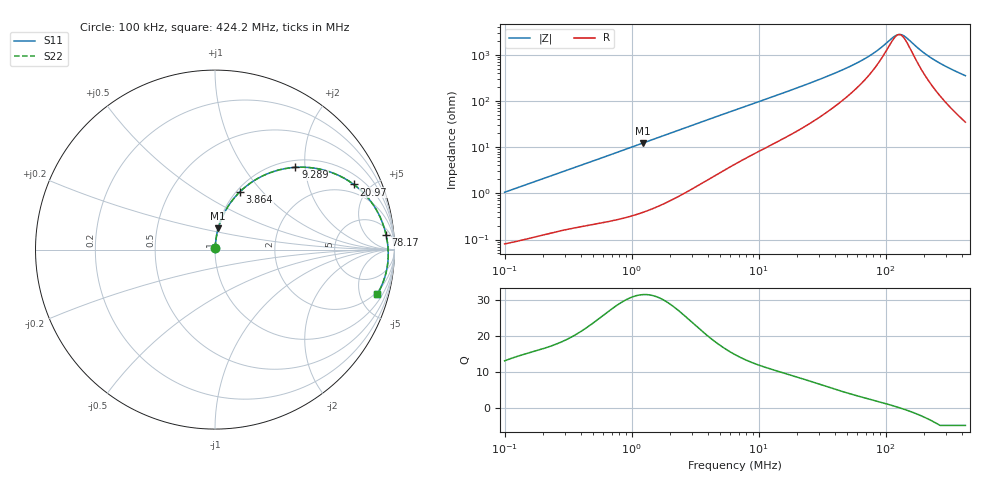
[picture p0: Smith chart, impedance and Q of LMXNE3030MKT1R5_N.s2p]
! LMXNE3030MKT1R5_N  S-PARAMETER MODEL  ( General Type )
! Model Generated by TAIYO YUDEN Corporation (https://www.yuden.co.jp/en/)
! Version 1.0
! TAIYO YUDEN Control No. 191023NI43SB-FBB
! Copyright(c) 2019 TAIYO YUDEN CO.,LTD. All Rights Reserved.
! Product Description (link to TY-COMPAS)
! https://ds.yuden.co.jp/TYCOMPAS/or/detail?pn=LMXNE3030MKT1R5NN&u=M
! Products Name : Inductors
! Characteristics :
!  Inductance : 1.5 uH , SRF(min) : 95 MHz , DC Resistance(max) : 0.066 Ohm
!  Rated Current : Saturation :1700 mA , Temp Rise : 1600 mA (40 degC)
!  Case Size : 3.0 x 3.0 / 0.118 x 0.118 [mm/inch] , Thickness : 1.2 / 0.047 [mm/inch]
!  (Conditions: Temperature = 25 degC , DC Bias Current/Voltage = 0A / 0V)
! External Node Assignments :
!  1  o---GGG---o  2
! GND o---------o GND
! Frequency Range : 0.1MHz  -  424.248007MHz  [ 402 STEP ]
# MHz S RI R 50
! Freq[MHz].  S11 Real  S11 Imag  S21 Real  S21 Imag  S12 Real  S12 Imag  S22 Real  S22 Imag
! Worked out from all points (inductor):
!   401 points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, 100 kHz to 424.2 MHz, reference 50 ohm
!   read as one part in series: L = 1.66 uH near 104.3 kHz
!   highest Q = 31.6 at 1.225 MHz (marker M1), where L = 1.59 uH
!   self-resonance near 127.2 MHz
!   S11 on the Smith chart (normalised r, x): 100 kHz: 1.00, +0.02; 3.864 MHz: 1.04, +0.76; 9.289 MHz: 1.14, +1.78; 20.97 MHz: 1.48, +3.96; 78.17 MHz: 10, +19; 424.2 MHz: 1.69, -6.98
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0.1  0.000914 0.0105  0.9991 -0.0105  0.9991 -0.0105  0.000914 0.0105
0.40516  0.00358 0.0408  0.9964 -0.0408  0.9964 -0.0408  0.00358 0.0408
1.225423  0.0184 0.1194  0.9816 -0.1194  0.9816 -0.1194  0.0184 0.1194
1.641544  0.0308 0.1574  0.9692 -0.1574  0.9692 -0.1574  0.0308 0.1574
2.598793  0.0703 0.2369  0.9297 -0.2369  0.9297 -0.2369  0.0703 0.2369
3.864414  0.1385 0.3218  0.8615 -0.3218  0.8615 -0.3218  0.1385 0.3218
6.650878  0.307 0.4283  0.693 -0.4283  0.693 -0.4283  0.307 0.4283
9.289316  0.4483 0.4583  0.5517 -0.4583  0.5517 -0.4583  0.4483 0.4583
13.52778  0.6135 0.4411  0.3865 -0.4411  0.3865 -0.4411  0.6135 0.4411
20.97378  0.7732 0.3629  0.2268 -0.3629  0.2268 -0.3629  0.7732 0.3629
26.38981  0.8336 0.3093  0.1664 -0.3093  0.1664 -0.3093  0.8336 0.3093
49.37507  0.9262 0.1669  0.0738 -0.1669  0.0738 -0.1669  0.9262 0.1669
63.43608  0.9437 0.1182  0.0563 -0.1182  0.0563 -0.1182  0.9437 0.1182
78.1676  0.9534 0.081  0.0466 -0.081  0.0466 -0.081  0.9534 0.081
106.9209  0.9622 0.0287  0.0378 -0.0287  0.0378 -0.0287  0.9622 0.0287
123.7502  0.9644 0.00458  0.0356 -0.00458  0.0356 -0.00458  0.9644 0.00458
129.028  0.9648 -0.00236  0.0352 0.00236  0.0352 0.00236  0.9648 -0.00236
137.3698  0.9652 -0.0129  0.0348 0.0129  0.0348 0.0129  0.9652 -0.0129
191.8651  0.9629 -0.0719  0.0371 0.0719  0.0371 0.0719  0.9629 -0.0719
231.5354  0.9574 -0.1084  0.0426 0.1084  0.0426 0.1084  0.9574 -0.1084
310.1588  0.94 -0.1719  0.06 0.1719  0.06 0.1719  0.94 -0.1719
424.248  0.9038 -0.2493  0.0962 0.2493  0.0962 0.2493  0.9038 -0.2493
